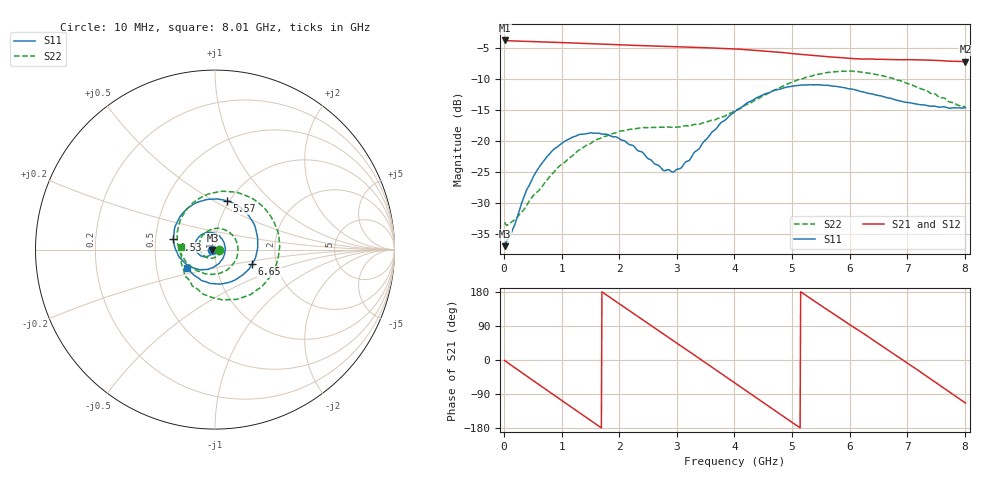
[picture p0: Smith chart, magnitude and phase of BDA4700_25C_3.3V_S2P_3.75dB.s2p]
!Agilent Technologies,E5071B,MY42404982,A.09.10
!Date: Mon Oct 20 18:04:33 2025
!Data & Calibration Information:
!Freq	S11:SOLT2(ON)	S21:SOLT2(ON)	S12:SOLT2(ON)	S22:SOLT2(ON)
# Hz S RI R 50
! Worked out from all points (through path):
!   801 points, 10 MHz to 8.01 GHz, reference 50 ohm
!   highest |S21| = -3.86 dB at 10 MHz (marker M1); lowest = -7.3 dB at 8.01 GHz (marker M2)
!   group delay of S21, straight-line fit = 288 ps
!   lowest |S11| = -36.9 dB at 10 MHz (marker M3), VSWR 1.03, Z = 48.6 - j0.15 ohm
!   |S11| at or under -10 dB: start of sweep to end of sweep
!   |S22| runs from -33.6 to -8.8 dB; largest |S21 - S12| = 0.0073
!   S11 on the Smith chart (normalised r, x): 10 MHz: 0.97, -0.00; 4.53 GHz: 0.62, +0.07; 5.57 GHz: 0.98, +0.57; 6.65 GHz: 1.49, -0.26; 8.01 GHz: 0.72, -0.15
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1e7  -0.0141 -0.00155  0.6408 -0.0137  0.6406 -0.0144  0.0221 -0.00181
3.3e8  -0.0225 -0.0253  0.5133 -0.3673  0.513 -0.3676  0.0202 -0.0185
7.2e8  -0.0598 -0.04  0.14 -0.6066  0.1404 -0.6065  -0.00726 -0.0463
1.02e9  -0.0943 -0.0217  -0.1971 -0.5836  -0.1969 -0.5839  -0.0509 -0.0413
1.35e9  -0.1105 0.0235  -0.4883 -0.3625  -0.4883 -0.3626  -0.086 0.0111
1.92e9  -0.0546 0.093  -0.5457 0.234  -0.5463 0.2338  -0.0131 0.1146
2.31e9  0.00923 0.0839  -0.2582 0.5238  -0.2583 0.5239  0.0869 0.0908
2.68e9  0.0514 0.037  0.1224 0.5642  0.1209 0.5635  0.1285 -0.00495
2.95e9  0.0549 -0.0132  0.3694 0.4362  0.3683 0.4351  0.103 -0.0765
3.36e9  0.0142 -0.083  0.5585 0.0697  0.5593 0.0697  0.00844 -0.1348
3.67e9  -0.0546 -0.1108  0.5028 -0.2371  0.5024 -0.2389  -0.0777 -0.1258
4.01e9  -0.1466 -0.09  0.2653 -0.479  0.2662 -0.4778  -0.1592 -0.0706
4.53e9  -0.2316 0.0565  -0.2274 -0.4749  -0.2273 -0.4758  -0.2088 0.1052
4.94e9  -0.1788 0.2047  -0.4712 -0.1862  -0.4712 -0.1886  -0.1196 0.2632
5.35e9  -0.0275 0.2808  -0.4553 0.172  -0.4562 0.1691  0.0831 0.3223
5.57e9  0.0674 0.271  -0.3483 0.3244  -0.3488 0.3242  0.2016 0.2882
6.08e9  0.222 0.1321  0.0351 0.456  0.0363 0.4579  0.3576 0.0508
6.65e9  0.2065 -0.0816  0.3977 0.2125  0.3983 0.2117  0.237 -0.2228
6.68e9  0.2011 -0.0911  0.4079 0.191  0.4088 0.1902  0.2239 -0.2324
7.06e9  0.1017 -0.1741  0.4355 -0.1073  0.4351 -0.1083  0.0463 -0.28
7.46e9  -0.0232 -0.1887  0.2507 -0.3662  0.2503 -0.3664  -0.1205 -0.2069
8.01e9  -0.1539 -0.1021  -0.1728 -0.3964  -0.1715 -0.397  -0.1869 0.0139
